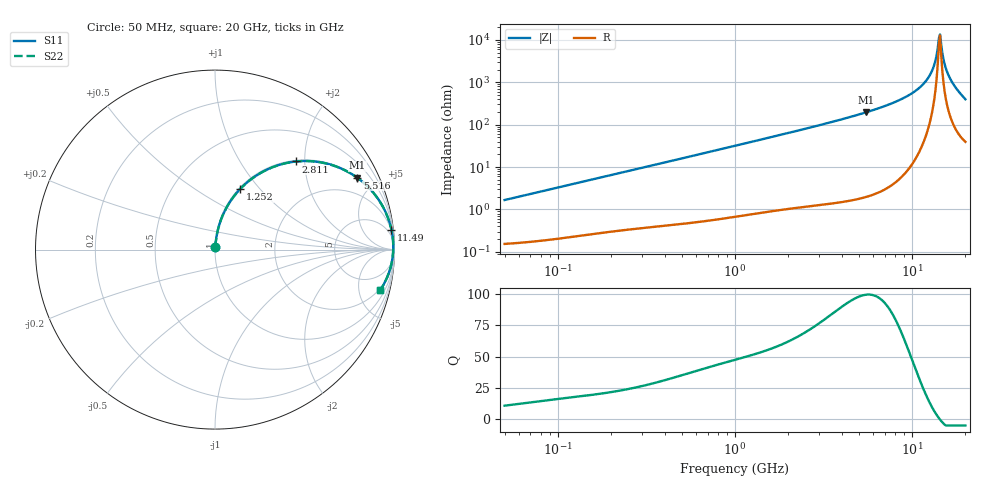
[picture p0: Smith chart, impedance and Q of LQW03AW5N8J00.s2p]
!Murata Part Number: LQW03AW5N8J00
!These Parameters are Measured in Series Mode Connection
!  o--[Z]--o
!Port1  Port2
!  o-------o
!Freq. Start=50[MHz] Stop=20[GHz], 401[Steps]
# Hz S RI R 50
!Freq.(Hz) S11(Real) S11(Imag) S21(Real) S21(Imag) S12(Real) S12(Imag) S22(Real) S22(Imag)
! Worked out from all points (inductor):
!   401 points, 50 MHz to 20 GHz, reference 50 ohm
!   read as one part in series: L = 5.27 nH near 51.52 MHz
!   highest Q = 99.6 at 5.516 GHz (marker M1), where L = 5.68 nH
!   self-resonance near 14.17 GHz
!   S11 on the Smith chart (normalised r, x): 50 MHz: 1.00, +0.03; 1.252 GHz: 1.02, +0.79; 2.811 GHz: 1.02, +1.82; 5.516 GHz: 1.04, +3.93; 11.49 GHz: 2, +18; 20 GHz: 1.79, -7.92
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5e7  0.0018 0.0165  0.9982 -0.0165  0.9982 -0.0165  0.0018 0.0165
1.364002e8  0.00438 0.0443  0.9956 -0.0443  0.9956 -0.0443  0.00438 0.0443
3.721004e8  0.0178 0.1165  0.9822 -0.1165  0.9822 -0.1165  0.0178 0.1165
1e9  0.0965 0.285  0.9035 -0.285  0.9035 -0.285  0.0965 0.285
1.251922e9  0.1413 0.3387  0.8587 -0.3387  0.8587 -0.3387  0.1413 0.3387
2.728004e9  0.4376 0.4893  0.5624 -0.4893  0.5624 -0.4893  0.4376 0.4893
2.810964e9  0.453 0.4911  0.547 -0.4911  0.547 -0.4911  0.453 0.4911
5.515528e9  0.7922 0.4007  0.2078 -0.4007  0.2078 -0.4007  0.7922 0.4007
7.442007e9  0.8987 0.2961  0.1013 -0.2961  0.1013 -0.2961  0.8987 0.2961
9.600142e9  0.9581 0.1914  0.0419 -0.1914  0.0419 -0.1914  0.9581 0.1914
1.149051e10  0.9831 0.1106  0.0169 -0.1106  0.0169 -0.1106  0.9831 0.1106
1.238412e10  0.9893 0.0749  0.0107 -0.0749  0.0107 -0.0749  0.9893 0.0749
1.295331e10  0.9917 0.0527  0.00828 -0.0527  0.00828 -0.0527  0.9917 0.0527
1.354865e10  0.993 0.0297  0.00695 -0.0297  0.00695 -0.0297  0.993 0.0297
1.396067e10  0.9933 0.014  0.00672 -0.014  0.00672 -0.014  0.9933 0.014
1.417136e10  0.9932 0.00598  0.00681 -0.00598  0.00681 -0.00598  0.9932 0.00598
1.438523e10  0.993 -0.00214  0.00705 0.00214  0.00705 0.00214  0.993 -0.00214
1.460232e10  0.9926 -0.0104  0.00744 0.0104  0.00744 0.0104  0.9926 -0.0104
1.550395e10  0.9893 -0.0446  0.0107 0.0446  0.0107 0.0446  0.9893 -0.0446
1.621653e10  0.9847 -0.0718  0.0153 0.0718  0.0153 0.0718  0.9847 -0.0718
1.774144e10  0.9682 -0.1313  0.0318 0.1313  0.0318 0.1313  0.9682 -0.1313
2e10  0.921 -0.2246  0.079 0.2246  0.079 0.2246  0.921 -0.2246
